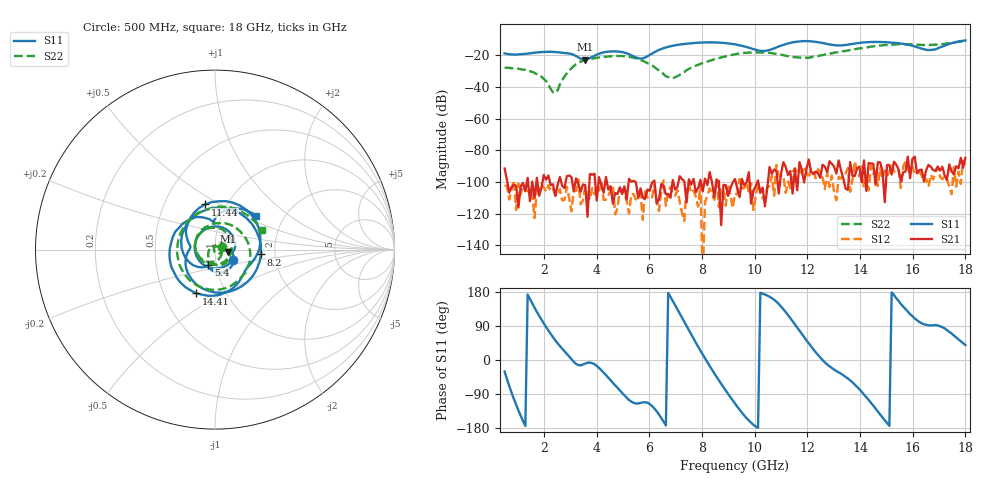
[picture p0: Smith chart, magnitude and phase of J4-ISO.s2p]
!Agilent Technologies,N5230A,MY45001360,A.07.50.67
!Agilent N5230A: A.07.50.67
!Date: Tuesday, April 16, 2024 15:55:22
!Correction: S11(Full 2 Port(1,2))
!S21(Full 2 Port(1,2))
!S12(Full 2 Port(1,2))
!S22(Full 2 Port(1,2))
!S2P File: Measurements: S11, S21, S12, S22:
# Hz S  dB  R 50
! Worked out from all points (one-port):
!   201 points, 500 MHz to 18 GHz, reference 50 ohm
!   lowest |S11| = -22.7 dB at 3.562 GHz (marker M1), VSWR 1.16, Z = 57.8 - j1.39 ohm
!   |S11| at or under -10 dB: start of sweep to end of sweep
!   S11 on the Smith chart (normalised r, x): 500 MHz: 1.21, -0.14; 5.4 GHz: 0.92, -0.16; 8.2 GHz: 1.69, -0.10; 11.44 GHz: 0.79, +0.43; 14.41 GHz: 0.73, -0.38; 18 GHz: 1.45, +0.59
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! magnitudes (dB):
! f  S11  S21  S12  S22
! 500 MHz  -18.8  -91.5  -102.3  -27.8
! 1.637 GHz  -18.3  -110.2  -122.8  -31.1
! 2.075 GHz  -17.8  -98.6  -106.1  -36.2
! 2.425 GHz  -17.9  -108.8  -108.2  -43.6
! 2.95 GHz  -18.8  -95.9  -110.0  -29.7
! 3.475 GHz  -22.6  -101.6  -111.7  -23.5
! 3.562 GHz  -22.7  -102.0  -103.3  -23.0
! 4.525 GHz  -17.5  -102.7  -105.2  -20.6
! 5.4 GHz  -20.6  -99.3  -107.7  -21.5
! 5.75 GHz  -21.9  -110.0  -124.0  -23.5
! 6.362 GHz  -16.5  -111.0  -118.4  -29.5
! 6.888 GHz  -13.9  -98.8  -107.1  -34.3
! 8.2 GHz  -11.8  -102.0  -108.8  -23.9
! 9.25 GHz  -13.0  -98.2  -107.4  -19.4
! 10.39 GHz  -17.2  -115.4  -111.5  -18.3
! 11.44 GHz  -11.8  -107.4  -93.3  -21.1
! 12.22 GHz  -11.3  -95.0  -91.6  -20.9
! 13.19 GHz  -13.8  -86.4  -96.7  -18.0
! 14.41 GHz  -11.5  -88.4  -89.8  -14.5
! 15.11 GHz  -11.9  -89.3  -93.6  -13.4
! 16.6 GHz  -16.7  -89.2  -103.0  -13.5
! 18 GHz  -10.6  -84.7  -89.3  -11.0
